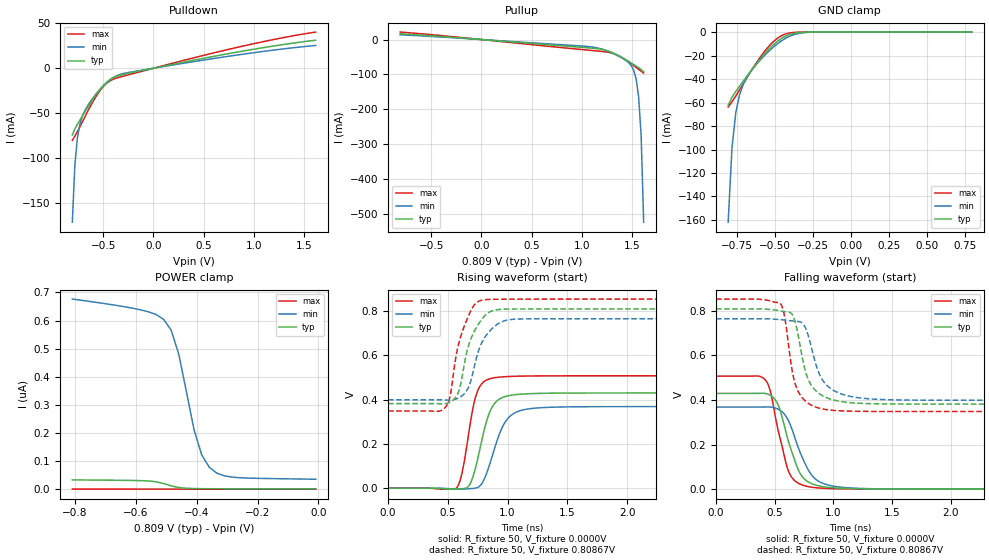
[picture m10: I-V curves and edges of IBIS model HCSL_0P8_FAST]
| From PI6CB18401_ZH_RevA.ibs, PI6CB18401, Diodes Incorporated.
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[Model]   HCSL_0P8_FAST
Model_type Output
Vref=0.8000V
Vmeas=900mV
| variable   typ   min   max
C_comp   2.000pF   1.970pF   2.030pF
[Voltage Range]   0.80867V   0.76428V   0.85294V
[POWER Clamp Reference]   0.80867V   0.76428V   0.85294V
[GND Clamp Reference]   0.0000V   0.0000V   0.0000V
[Pullup Reference]   0.80867V   0.76428V   0.85294V
[Pulldown Reference]   0.0000V   0.0000V   0.0000V
[Temperature Range]   25   85   -40
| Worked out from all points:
|   slope of the pulldown table from 0 to 0.121 V, typ, clamps not added: 43.9 ohm
|   slope of the pullup table from 0 to 0.121 V, typ, clamps not added: 43.9 ohm
|   GND clamp passes 1 mA (typ) near -0.37 V on its own axis
|   falling waveform, R_fixture 50, V_fixture 0.0000V: 20-80 % time 149ps typ, 172ps min, 127ps max; typ from 0.43 V to 0 V
|   rising waveform, R_fixture 50, V_fixture 0.0000V: 20-80 % time 122ps typ, 147ps min, 98.2ps max; typ from 0 V to 0.43 V
|   falling waveform, R_fixture 50, V_fixture 0.80867V: 20-80 % time 124ps typ, 149ps min, 99.5ps max; typ from 0.809 V to 0.382 V
|   rising waveform, R_fixture 50, V_fixture 0.80867V: 20-80 % time 131ps typ, 138ps min, 123ps max; typ from 0.382 V to 0.809 V
[GND Clamp]
| Voltage   I(typ)   I(min)   I(max)
-808.7mV  -62.12mA   -161.9mA   -63.86mA
-783.7mV  -55.6mA    -98.8mA    -59.36mA
-758.7mV  -50.64mA   -68.72mA   -54.46mA
-733.7mV  -46.08mA   -53.26mA   -49.26mA
-708.7mV  -41.61mA   -44.26mA   -43.9mA
-658.7mV  -32.83mA   -33.35mA   -33.29mA
-558.7mV  -16.95mA   -18.51mA   -14.73mA
-483.7mV  -7.773mA   -9.828mA   -5.14mA
-408.7mV  -2.206mA   -3.768mA   -815.3uA
-358.7mV  -647.7uA   -1.514mA   -143.2uA
-283.7mV  -64.34uA   -253.4uA   -5.991uA
791.3mV   1.208nA    35.61nA    1.246pA
[POWER Clamp]
| Voltage   I(typ)   I(min)   I(max)
-808.7mV  33.02nA    676.5nA    257.7pA
-583.7mV  30.32nA    637.8nA    188.8pA
-533.7mV  26.33nA    621.5nA    64.6pA
-508.7mV  20.08nA    604.6nA    40.81pA
-483.7mV  11.74nA    565.4nA    32.71pA
-458.7mV  5.847nA    479.8nA    29.42pA
-408.7mV  2.125nA    211.3nA    26.04pA
-383.7mV  1.712nA    122.8nA    24.68pA
-358.7mV  1.545nA    77.92nA    23.35pA
-333.7mV  1.471nA    57.06nA    22.03pA
-258.7mV  1.389nA    40.71nA    18.09pA
-8.67mV   1.225nA    35.32nA    4.944pA
[Pulldown]
| Voltage   I(typ)   I(min)   I(max)
-808.7mV  -74.27mA   -171.4mA   -80.33mA
-783.7mV  -67.64mA   -108.2mA   -75.67mA
-758.7mV  -62.54mA   -78.03mA   -70.61mA
-733.7mV  -57.85mA   -62.46mA   -65.22mA
-683.7mV  -48.67mA   -47.13mA   -54.12mA
-633.7mV  -39.76mA   -37.93mA   -43.34mA
-533.7mV  -23.94mA   -23.52mA   -25.04mA
-433.7mV  -12.87mA   -12.77mA   -14.02mA
-308.7mV  -7.139mA   -6.169mA   -9.062mA
116.3mV   2.651mA    2.176mA    3.424mA
966.3mV   20.53mA    16.79mA    26.52mA
1.616V    31.19mA    25.32mA    40.23mA
[Pullup]
| Voltage   I(typ)   I(min)   I(max)
-808.7mV  16.57mA    13.58mA    21.32mA
1.091V    -24.38mA   -20.82mA   -31.08mA
1.191V    -27.61mA   -26.52mA   -33.84mA
1.291V    -35.78mA   -37.17mA   -38.25mA
1.366V    -45.82mA   -47.55mA   -46.33mA
1.441V    -58.07mA   -60.28mA   -58.88mA
1.491V    -66.98mA   -74.13mA   -68.92mA
1.516V    -71.53mA   -87.43mA   -74.27mA
1.541V    -76.11mA   -112.5mA   -79.76mA
1.566V    -80.77mA   -164.2mA   -85.31mA
1.591V    -85.8mA    -275.9mA   -90.8mA
1.616V    -92.3mA    -522.6mA   -96.1mA
[Falling Waveform]
R_fixture = 50
V_fixture = 0.0000V
V_fixture_min = 0.0000V
V_fixture_max = 0.0000V
|   Time   V(typ)   V(min)   V(max)
0s        429.6mV    368.3mV    507.1mV
420ps     429.3mV    368.9mV    490.1mV
460ps     422.1mV    368.8mV    445.4mV
530ps     377.4mV    358.6mV    261.9mV
620ps     208.9mV    304.6mV    77.4mV
710ps     76.73mV    173.6mV    24.32mV
790ps     31.2mV     82.65mV    11.1mV
920ps     10.59mV    24.18mV    3.861mV
1.24ns    1.373mV    3.189mV    491.2uV
5ns       22.08uV    23.42uV    20.81uV
[Rising Waveform]
R_fixture = 50
V_fixture = 0.0000V
V_fixture_min = 0.0000V
V_fixture_max = 0.0000V
|   Time   V(typ)   V(min)   V(max)
0s        10.31uV    10.88uV    10.31uV
570ps     -3.321mV   -3.915mV   9.813uV
620ps     -1.938mV   -3.699mV   71.94mV
670ps     6.851mV    -2.606mV   231.4mV
740ps     110.5mV    1.848mV    425.2mV
800ps     253.1mV    35.87mV    479.7mV
880ps     374.2mV    160.1mV    497.3mV
1.01ns    417.5mV    319.3mV    503.8mV
1.22ns    426.9mV    360.7mV    506.3mV
5ns       429.6mV    368.3mV    507.1mV
[Falling Waveform]
R_fixture = 50
V_fixture = 0.80867V
V_fixture_min = 0.76428V
V_fixture_max = 0.85294V
|   Time   V(typ)   V(min)   V(max)
0s        808.7mV    764.3mV    852.9mV
550ps     799.7mV    760.7mV    831.6mV
590ps     796.1mV    758.6mV    756.3mV
640ps     789.6mV    755.6mV    559.7mV
690ps     716.3mV    753mV      450mV
780ps     499.8mV    698.5mV    387.4mV
910ps     418.6mV    487.4mV    359.7mV
1.08ns    392mV      425.2mV    351.2mV
1.38ns    383.1mV    403mV      348.7mV
5ns       381.6mV    398.7mV    348.2mV
[Rising Waveform]
R_fixture = 50
V_fixture = 0.80867V
V_fixture_min = 0.76428V
V_fixture_max = 0.85294V
|   Time   V(typ)   V(min)   V(max)
0s        381.5mV    398.7mV    348.2mV
480ps     381.2mV    397.9mV    365mV
520ps     388.3mV    397.7mV    417.4mV
570ps     413.7mV    402.8mV    599.8mV
620ps     504mV      417.5mV    704.8mV
680ps     654.4mV    464.1mV    786.1mV
790ps     765.3mV    662.6mV    848.5mV
920ps     805.4mV    741.4mV    852.2mV
1.08ns    808.1mV    762.7mV    852.5mV
5ns       808.6mV    764.3mV    852.9mV
[Ramp]
| variable   typ   min   max
dV/dt_r   0.25792V/122.44p   0.22123V/146.81p   0.30444V/98.301p
dV/dt_f   0.25615V/123.99p   0.21902V/149.08p   0.30272V/99.498p
R_load = 50
